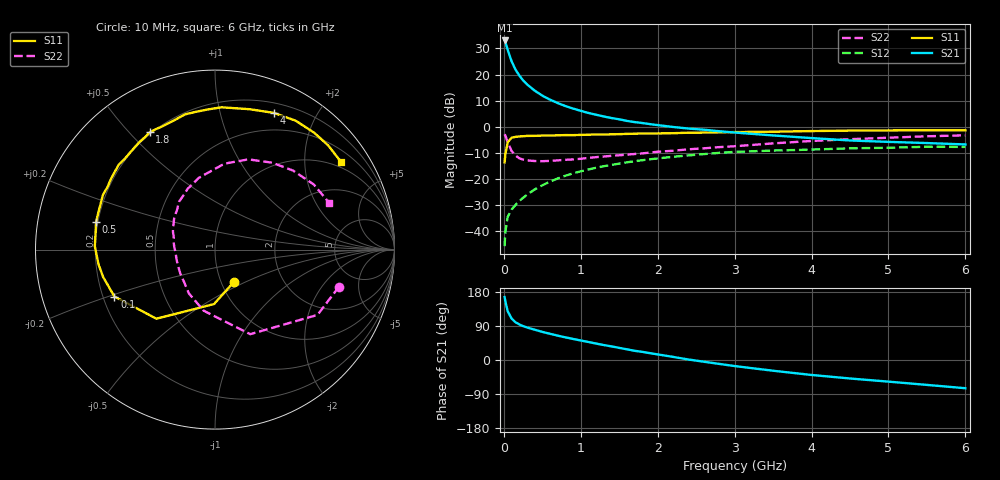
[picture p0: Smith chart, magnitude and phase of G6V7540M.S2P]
! SIEMENS Small Signal Semiconductors
! BFG193
! Si NPN RF Bipolar Junction Transistor in SOT223
! VCE = 0.75 V  IC = 40 mA
! Common Emitter S-Parameters:  August  1996
# GHz  S  MA  R  50
!  f  S11  S21  S12  S22
! GHz  MAG  ANG  MAG  ANG  MAG  ANG  MAG  ANG
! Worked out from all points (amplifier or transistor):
!   36 points, 10 MHz to 6 GHz, reference 50 ohm
!   highest |S21| = 33.1 dB at 10 MHz (marker M1)
!   |S21| within 3 dB of that: start of sweep to 44.01 MHz
!   unconditionally stable (mu >= 1): 244.8 MHz to end of sweep
!   at 250 MHz: K = 1.01, MAG = 22.0 dB, |S12| = -27.2 dB
!   at 1.4 GHz: K = 1.14, MAG = 6.7 dB, |S12| = -14.6 dB
!   at 6 GHz: K = 1.04, MAG = -0.7 dB, |S12| = -7.7 dB
!   S11 on the Smith chart (normalised r, x): 10 MHz: 1.15, -0.43; 100 MHz: 0.25, -0.21; 500 MHz: 0.19, +0.11; 1.8 GHz: 0.19, +0.57; 4 GHz: 0.30, +1.48; 6 GHz: 0.82, +2.98
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0.01  0.2087 -59.8  44.96 166.1  0.0052 75.1  0.7212 -16.6
0.02  0.3034 -91.0  41.5 154.3  0.0099 70.7  0.6773 -32.5
0.05  0.5048 -130.3  29.79 128.6  0.0188 56.3  0.5104 -67.4
0.1  0.6185 -155.0  18.07 109.7  0.026 52.7  0.3462 -100.5
0.15  0.6419 -166.3  12.55 99.8  0.0318 53.8  0.2843 -120.8
0.2  0.6536 -172.6  9.651 94.0  0.038 56.6  0.2505 -133.1
0.25  0.6611 -177.7  7.749 89.5  0.0438 58.6  0.236 -144.5
0.3  0.6697 178.5  6.516 85.9  0.0502 60.6  0.2283 -151.6
0.4  0.6716 172.4  4.933 80.0  0.0632 61.2  0.2215 -163.9
0.5  0.68 167.0  3.955 74.2  0.0759 60.7  0.2201 -172.6
0.6  0.6821 162.1  3.308 69.2  0.0892 60.0  0.2226 -178.8
0.8  0.6951 153.8  2.499 59.8  0.1157 56.6  0.2339 169.9
1.1  0.7062 142.4  1.841 47.5  0.1526 50.9  0.2543 157.1
1.4  0.7181 131.4  1.473 35.9  0.1866 43.7  0.2784 145.6
1.8  0.7476 119.1  1.183 21.5  0.2296 34.2  0.3102 132.3
2.2  0.7548 107.8  0.994 8.2  0.2672 23.8  0.3484 120.6
2.8  0.7832 92.1  0.823 -10.3  0.3176 8.9  0.4089 103.0
3.5  0.8057 76.1  0.684 -28.3  0.3515 -9.1  0.4818 83.7
4  0.8293 66.7  0.609 -39.5  0.3665 -18.6  0.5361 69.7
4.5  0.8472 58.0  0.548 -48.8  0.388 -28.4  0.5795 56.7
5.5  0.8572 42.6  0.489 -65.7  0.4154 -50.2  0.6591 33.4
6  0.8552 34.9  0.46 -74.5  0.4126 -62.7  0.6878 22.2
